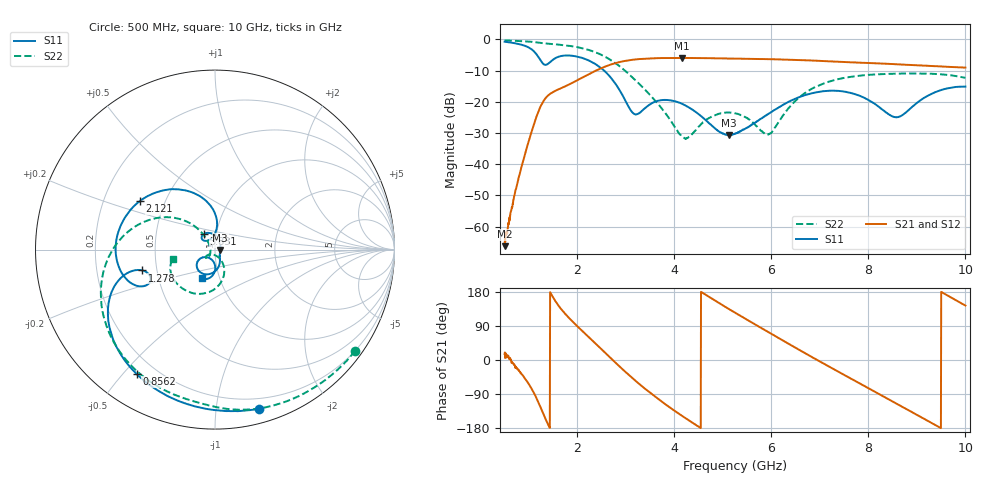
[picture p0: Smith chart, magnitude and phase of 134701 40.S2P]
!  2-Port S-parameters saved by WinCal
! VAR MeasName=S-Parameters (CALIBRATED_DATA) read from VNA (N5242A)
! VAR MeasDate=2013-7-3 16:37:29
! VAR NAME=134701 40
! VAR FILENAME=134701 40.S2P
! VAR DATE=2013-7-3 16:37:29
! VAR PHYS_PORTS=1,2
# Hz S MA R 50
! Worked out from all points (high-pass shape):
!   1601 points, 500 MHz to 10 GHz, reference 50 ohm
!   highest |S21| = -5.92 dB at 4.157 GHz (marker M1); lowest = -66.3 dB at 500 MHz (marker M2)
!   |S21| within 3 dB of the highest: 2.539 GHz to 9.831 GHz (7.293 GHz wide, 118 % of centre)
!   lowest |S11| = -30.7 dB at 5.125 GHz (marker M3), VSWR 1.06, Z = 53 - j0.437 ohm
!   |S11| at or under -10 dB: 2.551 GHz to end of sweep
!   |S22| runs from -31.9 to -0.3 dB; largest |S21 - S12| = 0.0017
!   S11 on the Smith chart (normalised r, x): 500 MHz: 0.11, -1.31; 856.2 MHz: 0.13, -0.54; 1.278 GHz: 0.41, -0.12; 2.121 GHz: 0.36, +0.26; 3.831 GHz: 0.87, +0.15; 10 GHz: 0.82, -0.27
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5e8  0.92 -74.6  0.0004841 15.6  0.0005845 20.0  0.9627 -35.9
8.5625e8  0.8189 -122.3  0.009507 -38.5  0.009487 -38.4  0.9394 -61.2
1.064062e9  0.6874 -150.3  0.03482 -77.4  0.03472 -77.9  0.9147 -76.1
1.277812e9  0.4206 -164.0  0.09561 -135.9  0.09548 -136.1  0.8724 -91.0
1.550938e9  0.5028 -158.1  0.1506 154.6  0.1501 154.4  0.8338 -108.8
2.085312e9  0.5096 150.8  0.2409 78.4  0.2396 78.4  0.7276 -148.0
2.120938e9  0.4987 147.3  0.2488 74.1  0.2478 74.1  0.7168 -150.8
2.483125e9  0.3503 113.1  0.3431 30.2  0.3416 30.3  0.5718 -179.7
2.880938e9  0.1489 85.6  0.4356 -18.4  0.4351 -18.4  0.3667 151.2
3.189688e9  0.06298 115.6  0.4768 -53.9  0.4769 -53.9  0.2251 135.5
3.670625e9  0.104 134.7  0.502 -103.3  0.5009 -103.2  0.09104 128.3
3.830938e9  0.1071 125.7  0.5038 -118.3  0.504 -118.3  0.06324 131.3
4.1575e9  0.09259 102.7  0.5056 -147.4  0.5047 -147.3  0.02776 167.4
5.125312e9  0.02916 -8.1  0.4943 134.5  0.4944 134.4  0.06718 -138.4
5.25e9  0.03087 -25.9  0.4924 124.9  0.4923 125.0  0.06561 -141.1
5.950625e9  0.06524 -65.0  0.4825 72.7  0.4824 72.7  0.03035 -98.1
6.835312e9  0.1368 -100.6  0.4589 7.8  0.4594 7.8  0.1621 -73.5
7.660625e9  0.1372 -137.9  0.4288 -50.6  0.4296 -50.7  0.2529 -104.5
8.420625e9  0.06288 -137.4  0.406 -104.0  0.4045 -104.0  0.2802 -126.7
8.658125e9  0.05856 -109.0  0.3962 -120.8  0.3967 -120.7  0.2834 -132.5
9.228125e9  0.1254 -91.4  0.3774 -161.0  0.3775 -160.8  0.2826 -146.5
1e10  0.1753 -114.6  0.3535 143.7  0.3533 143.7  0.2418 -167.5
